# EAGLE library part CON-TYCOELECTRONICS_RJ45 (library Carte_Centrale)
CORCOM Modular RJ Jacks No Shield Source: www.tycoelectronics.com .. ENG_DS_1654001_1099_RJ_L_0507.pdf
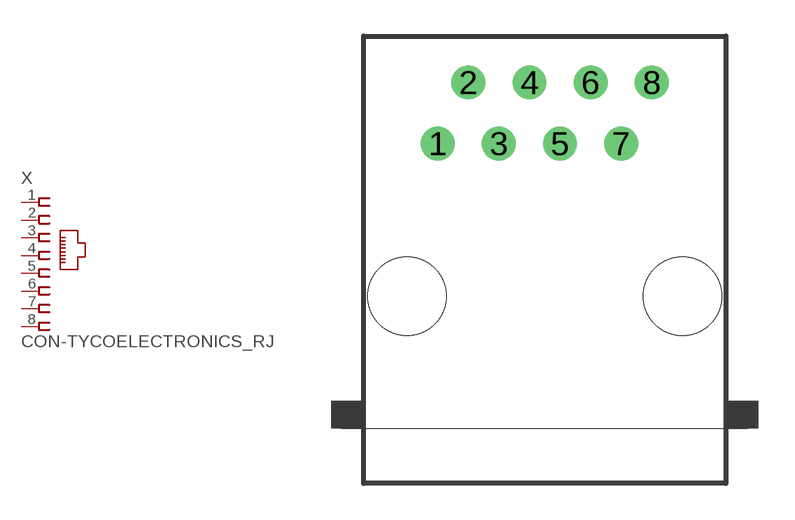
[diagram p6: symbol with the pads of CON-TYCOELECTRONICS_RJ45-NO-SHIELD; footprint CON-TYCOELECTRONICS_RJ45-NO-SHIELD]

Designator prefix X

## CON-TYCOELECTRONICS_RJ45, CON-TYCOELECTRONICS_RJ45-6L-B (MPN: RJ45-6L-B; OC_FARNELL: unknown; OC_NEWARK: 16R6090), CON-TYCOELECTRONICS_RJ45-6L-S (MPN: RJ45-6L-S; OC_FARNELL: unknown; OC_NEWARK: 16R6091), CON-TYCOELECTRONICS_RJ45-6X (MPN: RJ45-6X; OC_FARNELL: unknown; OC_NEWARK: 01P1604), CON-TYCOELECTRONICS_RJ45-8L-B (MF: TYCO ELECTRONICS; MPN: RJ45-8L-B; OC_FARNELL: 1279843; OC_NEWARK: 52K4445), CON-TYCOELECTRONICS_RJ45-8L-S (MF: TYCO ELECTRONICS; MPN: RJ45-8L-S; OC_FARNELL: unknown; OC_NEWARK: 80K9067), CON-TYCOELECTRONICS_RJ45-8X (MPN: RJ45-8X; OC_FARNELL: unknown; OC_NEWARK: 16R6101)  [CON-TYCOELECTRONICS_RJ45-NO-SHIELD]
1  1  pas
2  2  pas
3  3  pas
4  4  pas
5  5  pas
6  6  pas
7  7  pas
8  8  pas

## Footprint CON-TYCOELECTRONICS_RJ45-NO-SHIELD (pad centres in mm)
RJ45 Low Profile No Shield For all RJ45 N and Z Series Models Source: www.tycoelectronics.com .. ENG_DS_1654001_1099_RJ_L_0507.pdf
drill 0.9 pad 1.4: 1 -4.445,6.35; 2 -3.175,8.89; 3 -1.905,6.35; 4 -0.635,8.89; 5 0.635,6.35; 6 1.905,8.89; 7 3.175,6.35; 8 4.445,8.89
hole 3.251 at -5.715,0
hole 3.251 at 5.715,0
